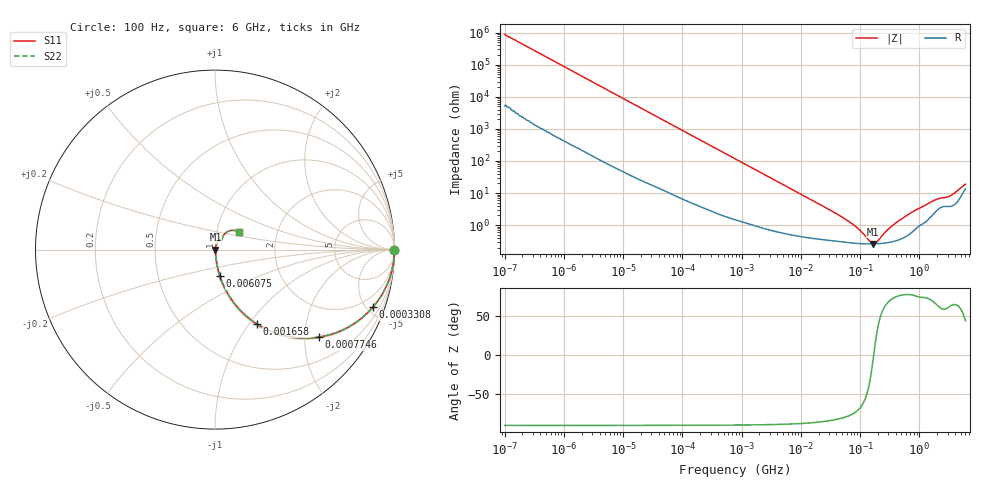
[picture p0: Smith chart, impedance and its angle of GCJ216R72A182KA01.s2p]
!Murata Part Number: GCJ216R72A182KA01
!These Parameters are Measured in Series Mode Connection
!Data Generated on Mar 13, 2026
!  o--ll--o
!Port1  Port2
!  o------o
!Operation Temp=25[degC], DC Bias Voltage=0[V]
!Freq. Start=100[Hz] Stop=6[GHz] 401[Steps]
# Hz S RI R 50
!Freq.(Hz) S11(Real) S11(Imag) S21(Real) S21(Imag) S12(Real) S12(Imag) S22(Real) S22(Imag)
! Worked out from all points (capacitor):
!   401 points, 100 Hz to 6 GHz, reference 50 ohm
!   read as one part in series: C = 1.81 nF near 109 Hz
!   lowest |Z| = 262 mohm at 166.9 MHz (marker M1)
!   series resonance near 170 MHz, so ESL is about 480 pH
!   S11 on the Smith chart (normalised r, x): 100 Hz: open; 330.8 kHz: 1.05, -5.45; 774.6 kHz: 1.03, -2.34; 1.658 MHz: 1.02, -1.10; 6.075 MHz: 1.01, -0.30; 6 GHz: 1.27, +0.26
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100  1 -0.000114  7e-07 0.000114  7e-07 0.000114  1 -0.000114
2008  1 -0.00227  1.62e-05 0.00227  1.62e-05 0.00227  1 -0.00227
40335  0.9977 -0.045  0.00232 0.045  0.00232 0.045  0.9977 -0.045
123542  0.9804 -0.1348  0.0196 0.1348  0.0196 0.1348  0.9804 -0.1348
330837  0.8791 -0.3213  0.1209 0.3213  0.1209 0.3213  0.8791 -0.3213
495019  0.7668 -0.4176  0.2332 0.4176  0.2332 0.4176  0.7668 -0.4176
774597  0.5767 -0.4878  0.4233 0.4878  0.4233 0.4878  0.5767 -0.4878
1108252  0.4031 -0.4832  0.5969 0.4832  0.5969 0.4832  0.4031 -0.4832
1658239  0.2357 -0.4158  0.7643 0.4158  0.7643 0.4158  0.2357 -0.4158
2967816  0.0921 -0.2779  0.9079 0.2779  0.9079 0.2779  0.0921 -0.2779
6075234  0.0273 -0.1466  0.9727 0.1466  0.9727 0.1466  0.0273 -0.1466
1.555665e7  0.00734 -0.0588  0.9927 0.0588  0.9927 0.0588  0.00734 -0.0588
6.817316e7  0.00293 -0.0118  0.9971 0.0118  0.9971 0.0118  0.00293 -0.0118
9.326766e7  0.00271 -0.00724  0.9973 0.00724  0.9973 0.00724  0.00271 -0.00724
1.459435e8  0.0026 -0.00175  0.9974 0.00175  0.9974 0.00175  0.0026 -0.00175
1.669249e8  0.0026 -0.000206  0.9974 0.000206  0.9974 0.000206  0.0026 -0.000206
1.909225e8  0.00263 0.00134  0.9974 -0.00134  0.9974 -0.00134  0.00263 0.00134
3.124326e8  0.00295 0.00744  0.997 -0.00744  0.997 -0.00744  0.00295 0.00744
8.366708e8  0.00782 0.0271  0.9922 -0.0271  0.9922 -0.0271  0.00782 0.0271
1.873145e9  0.028 0.0533  0.972 -0.0533  0.972 -0.0533  0.028 0.0533
3.352442e9  0.0417 0.0673  0.9583 -0.0673  0.9583 -0.0673  0.0417 0.0673
6e9  0.1317 0.0991  0.8683 -0.0991  0.8683 -0.0991  0.1317 0.0991
